(* This function block implements IEC 60870-5-101 master services *)
FUNCTION_BLOCK FB_IEC870_5_101MServices
VAR_IN_OUT
	stProcData 		: ST_IEC870_5_101MProcData;(* Process data send to or received from IEC 60870-5-101 slave device *)
	sysPara 		: ST_IEC870_5_101MSysPara; (* System parameters (data acquisition cycle times, common asdu address...) *)
	buffer			: ST_IEC870_5_101TBuffer; (* RX/TX buffer *)
	fbClock			: FB_LocalSystemTime;(* Internal clock: Local windows system time *)
	fbLog			: FB_IEC870_DebugLogFifo;(* Simple log buffer. We store/log here all our received slave data and other messages (for demonstration purpose only) *)
	bReset			: BOOL;(* Rising edge at this input resets service execution *)
END_VAR
VAR
	eState			: E_IEC870_5_101MState := e101MState_Init;(* Service/device execution state *)
	fbBuffer		: FB_IEC870_5_101TBufferCtrl;(* TX/RX buffer control function block *)
	txAsdu 			: ST_IEC870_5_101AOGen; (* Temp. asdu to send *)
	rxAsdu 			: ST_IEC870_5_101AOGen; (* Temp. received asdu *)
	
	fbTestTimer 	: TON;(* Test command cycle timer *)
	fbClockTimer	: TON;(* Clock synchronisation command cycle timer *)
	fbGeninTimer	: TON;(* General interrogation command cycle timer *)
	fbCoroTimer		: TON;(* Counter interrogation command cycle timer *)
	fbConTimer		: TON;(* Command activation confirmation timeout timer *)
	fbTermTimer		: TON;(* Command activation termination timeout timer *)
	
	bEndOfInit 		: BOOL;(* FALSE => Initialization in progress (first clock sync, general interrogation, counter interrogation... ), TRUE => End of initialization *)
	bTestConWait 	: BOOL;(* TRUE => Waiting for test command activation confirmation *)
	bClockConWait 	: BOOL;(* TRUE => Wating for clock synchronisation activation confirmation *)
	bGeninConWait	: BOOL;(* TRUE => Waiting for general interrogation activation confirmation *)
	bGeninTermWait	: BOOL;(* TRUE => Waiting for general interrogation activation termination *)
	bCoroConWait	: BOOL;(* TRUE => Waiting for counter interrogation activation confirmation *)
	bCoroTermWait	: BOOL;(* TRUE => Waiting for counter interrogation activation termination *)
	bCmdConWait		: BOOL;(* TRUE => Wating for command activation confirmation *)
	bCmdTermWait	: BOOL;(* TRUE => Waiting for command activation termination *)
	(* Temporary variables *)
	tT16			: T_CP16Time2a;(* 16 bit time tag value *)
	tT24			: T_CP24Time2a;(* 24 bit time tag value *)
	tT56			: T_CP56Time2a;(* 56 bit time tag value *)
	tT56_old		: T_CP56Time2a;(* 56 bit time tag value *)
	tT56_new		: T_CP56Time2a;(* 56 bit time tag value *)
	nCoi			: BYTE;(* Cause of initialization + LPC *)
	eCoi			: E_IEC870_5_101COI;(* Cause of initialization as enumerated type *)
	bLpc			: BOOL;(* Local parameter changed *)
	nFbp			: WORD := 16#55AA;(* Test command frame bit pattern activation data *)
	stSiq			: ST_IEC870_5_101SIQ;(* Single point information + quality descriptor *)
	stDiq			: ST_IEC870_5_101DIQ;(* Double point information + quality descriptor *)
	stQds			: ST_IEC870_5_101QDS;(* Measured value quality descriptor *)
	stQcr			: ST_IEC870_5_101QCR;(* Binary counter quality descriptor *)
	stQdp			: ST_IEC870_5_101QDP;(* Quality descriptor for events of protection equipment *)
	stSep			: ST_IEC870_5_101SEP;(* Quality descriptor for events of protection equipment *)
	stSpe			: ST_IEC870_5_101SPE;(* Start events of protection equipment *)
	stOci			: ST_IEC870_5_101OCI;(* Output cirquit information of protection equipment *)
	nVti			: BYTE;(* Value with transient state indication *)
	nBsi			: DWORD;(* Bitstring information *)
	nNva			: WORD;(* Normalized value *)
	nSva			: INT;(* Scalled value *)
	fR32			: REAL;(* Short floating point value *)
	nBcr			: DINT;(* Binary counter reading *)
	nScd			: DWORD;(* Status change detection *)
	nSco			: BYTE;(* Single command + qualifier *)
	nDco			: BYTE;(* Double  command + qualifier *)
	nRco			: BYTE;(* Regulating step command + qualifier *)
	nQos			: BYTE;(* Qualifier of setpoint command *)
	nQpm			: BYTE;(* Qualifier of parameter loading command *)
	nQpa			: BYTE;(* Qualifier of parameter activation command *)
	nQcc			: BYTE;(* Qualifier of counter interrogation command *)
	eFrz			: E_IEC870_5_101FRZ := eIEC870_FRZ_READ;
	nQoi			: BYTE;(* Qualifier of interrogation command *)
END_VAR

(* Please don't use the SIZEOF operator with CP56Time2a or CP24Time2a data type.
Because of the data alignment SIZEOF( tT56 ) or SIZEOF( tT24 ) leads to incorrect size. *)

IF bReset THEN(* Reset service execution *)
	bReset 	:= FALSE;
	eState 	:= e101MState_Init;
END_IF

(*-----------------------------------------------------------------------------------------*)
(* Generate new TX data (master requests) *)
(*-----------------------------------------------------------------------------------------*)
CASE eState OF
	e101MState_Init:(* Init state *)
		(* Reset all flags *)
		bEndOfInit 		:= FALSE;
		bTestConWait 	:= FALSE;
		bClockConWait	:= FALSE;
		bGeninConWait 	:= FALSE;
		bGeninTermWait	:= FALSE;
		bCoroConWait	:= FALSE;
		bCoroTermWait	:= FALSE;
		bCmdConWait		:= FALSE;
		bCmdTermWait	:= FALSE;
		(* Reset all timer *)
		fbTestTimer( IN := FALSE );
		fbClockTimer( IN := FALSE );
		fbGeninTimer( IN := FALSE );
		fbCoroTimer( IN := FALSE );
		fbConTimer( IN := FALSE );
		fbTermTimer( IN := FALSE );
		eState := e101MState_CycleStart;
	(*-----------------------------------------------------------------------------------------*)
	e101MState_CycleStart:(* Start of scan cycle *)
		eState := e101MState_TestAct;
	(*-----------------------------------------------------------------------------------------*)
	e101MState_TestAct:(* Send test command activation *)
		fbTestTimer( IN := bEndOfInit AND sysPara.bTest, PT := sysPara.tTest );
		IF NOT bEndOfInit OR fbTestTimer.Q THEN
			fbTestTimer( IN := FALSE );(* Reset timer *)
			fbTestTimer( IN := sysPara.bTest );
			
			(* Create asdu *)
			txAsdu.ident.eType 		:= C_TS_NA_1;(* Test command *)
			txAsdu.ident.bSQ 		:= FALSE;
			txAsdu.ident.nObj 		:= 1;
			txAsdu.ident.eCOT 		:= eIEC870_COT_ACT;(* Command activation *)
			txAsdu.ident.nORG 		:= sysPara.nOrg;(* Set originator address *)
			txAsdu.ident.bPN 		:= FALSE;
			txAsdu.ident.bT 		:= FALSE;
			txAsdu.ident.eClass 	:= eIEC870_Class_1;(* Put to the high priority tx buffer *)
			txAsdu.ident.asduAddr 	:= sysPara.asduAddr;(* Set common asdu address *)
			txAsdu.info.objAddr		:= 0;(* Set information object address *)

			nFbp := 16#55AA;(* Fixed bit pattern (FBP = 16#55AA ) to send *)
			F_iecResetStream( 0, txAsdu.info.stream );(* Clear previous data (this sets the stream length = 0 *)
			F_iecCopyBufferToStream( ADR( nFbp ), SIZEOF( nFbp ), txAsdu.info.stream );(* Put test bit pattern to stream *)
			fbBuffer.TxAddObj( putObj := txAsdu, buffer := buffer, bOk=>bTestConWait );(* Put asdu to the TX fifo *)
			IF fbBuffer.bOk THEN(* Success *)
				fbLog.A_LogHint( sPut := CONCAT( '<=', IEC101ASDU_TO_STRING( txAsdu ) ) );(* Log data (for demonstration purpose only) *)
				fbConTimer( IN := FALSE );(* Reset timer *)
				eState := e101MState_TestCon;(* Wait for test command activation confirmation *)
			ELSE(* Report send buffer overflow warning *)
				fbLog.A_LogWarning( sPut := '::TX buffer overflow (test command)!' );(* Log warning *)
			END_IF
		ELSE(* Start clock synchronisation command activation *)
			eState := e101MState_ClockAct;		
		END_IF
	
	e101MState_TestCon:(* Wait for test command activation confirmation *)
		fbConTimer( IN := bTestConWait, PT := sysPara.tCon );(* Perform timeout measure *)
		IF fbConTimer.Q THEN(* Report test command confirmation timeout error *)
			fbConTimer( IN := FALSE );(* Reset timer *)
			fbLog.A_LogError( sPut := '::Activation confirmation timeout (test command)!' );(* Log error *)
			eState := e101MState_Init;
		ELSIF NOT bTestConWait THEN(* Start clock synchronisation command activation *)
			eState := e101MState_ClockAct;
		END_IF
	(*-----------------------------------------------------------------------------------------*)
	e101MState_ClockAct:(* Send clock synchronisation command *)
		fbClockTimer( IN := bEndOfInit AND sysPara.bClock, PT := sysPara.tClock );
		IF NOT bEndOfInit OR fbClockTimer.Q THEN
			fbClockTimer( IN := FALSE );(* Reset timer *)
			fbClockTimer( IN := sysPara.bClock );
			
			(* Create asdu *)
			txAsdu.ident.eType 		:= C_CS_NA_1;(* Clock synchronisation command *)
			txAsdu.ident.bSQ 		:= FALSE;
			txAsdu.ident.nObj 		:= 1;
			txAsdu.ident.eCOT 		:= eIEC870_COT_ACT;(* Command activation *)
			txAsdu.ident.nORG 		:= sysPara.nOrg;(* Set originator address *)
			txAsdu.ident.bPN 		:= FALSE;
			txAsdu.ident.bT 		:= FALSE;
			txAsdu.ident.eClass 	:= eIEC870_Class_1;(* Put to the high priority tx buffer *)
			txAsdu.ident.asduAddr 	:= sysPara.asduAddr;(* Set common asdu address *)
			txAsdu.info.objAddr		:= 0;(* Set information object address *)
			
			tT56_new				:= SYSTEMTIME_TO_CP56Time2a( fbClock.systemTime, SU := fbClock.tzID = eTimeZoneID_Daylight );(* Get current windows loacal system time in CP56Time2a format *)
			F_iecResetStream( 0, txAsdu.info.stream );(* Clear previous data (this sets the stream length = 0 *)
			F_iecCopyBufferToStream( ADR( tT56_new ), 7(* SIZEOF( tT56_new ) - 1 *), txAsdu.info.stream );(* Put new sync time to stream *)
			fbBuffer.TxAddObj( putObj := txAsdu, buffer := buffer, bOk=>bClockConWait );(* Put asdu to the TX fifo *)
			IF fbBuffer.bOk THEN(* Success *)
				fbLog.A_LogHint( sPut := CONCAT( '<=', IEC101ASDU_TO_STRING( txAsdu ) ) );(* Log data (for demonstration purpose only) *)
				fbConTimer( IN := FALSE );(* Reset timer *)
				eState := e101MState_ClockCon;(* Wait for clock synchronisation command activation confirmation *)
			ELSE(* Report send buffer overflow warning *)
				fbLog.A_LogWarning( sPut := '::TX buffer overflow (clock synchronisation command)!' );(* Log warning *)
			END_IF			
		ELSE(* Start general interrogation command activation *)
			eState := e101MState_GeninAct;
		END_IF

	e101MState_ClockCon:(* Wait for clock synchronisation command activation confirmation *)
		fbConTimer( IN := bClockConWait, PT := sysPara.tCon );(* Perform timeout measure *)
		IF fbConTimer.Q THEN(* Report command confirmation timeout error *)
			fbConTimer( IN := FALSE );(* Reset timer *)
			fbLog.A_LogError( sPut := '::Activation confirmation timeout (clock synchronisation command)!' );(* Log error *)
			eState := e101MState_Init;
		ELSIF NOT bClockConWait THEN(* Start general interrogation command activation *)
			eState := e101MState_GeninAct;
		END_IF
	(*-----------------------------------------------------------------------------------------*)
	e101MState_GeninAct:(* Send general interrogation command activation*)
		fbGeninTimer( IN := bEndOfInit AND sysPara.bGenin, PT := sysPara.tGenin );
		IF NOT bEndOfInit OR fbGeninTimer.Q THEN
			fbGeninTimer( IN := FALSE );(* Reset timer *)
			fbGeninTimer( IN := sysPara.bGenin );
			
			(* Create asdu *)
			txAsdu.ident.eType 		:= C_IC_NA_1;(* General interrogation command *)
			txAsdu.ident.bSQ 		:= FALSE;
			txAsdu.ident.nObj 		:= 1;
			txAsdu.ident.eCOT 		:= eIEC870_COT_ACT;(* Command activation *)
			txAsdu.ident.nORG 		:= sysPara.nOrg;(* Set originator address *)
			txAsdu.ident.bPN 		:= FALSE;
			txAsdu.ident.bT 		:= FALSE;
			txAsdu.ident.eClass 	:= eIEC870_Class_1;(* Put to the high priority tx buffer *)
			txAsdu.ident.asduAddr 	:= sysPara.asduAddr;(* Set common asdu address *)
			txAsdu.info.objAddr		:= 0;(* Set information object address *)
			
			nQoi	:= INT_TO_BYTE( sysPara.eGeninQoi );(* Qualifier of general interrogation command (QOI) to send *)
			F_iecResetStream( 0, txAsdu.info.stream );(* Clear previous data (this sets the stream length = 0 *)
			F_iecCopyBufferToStream( ADR( nQoi ), SIZEOF( nQoi ), txAsdu.info.stream );(* Put QOI to stream *)
			fbBuffer.TxAddObj( putObj := txAsdu, buffer := buffer, bOk=>bGeninConWait );(* Put asdu to the TX fifo *)
			IF fbBuffer.bOk THEN(* Success *)
				fbLog.A_LogHint( sPut := CONCAT( '<=', IEC101ASDU_TO_STRING( txAsdu ) ) );(* Log data (for demonstration purpose only) *)
				fbConTimer( IN := FALSE );(* Reset timer *)
				fbTermTimer( IN := FALSE );(* Reset timer *)
				bGeninTermWait := bGeninConWait;(* Wait for general interrogation activation termination too *)
				eState := e101MState_GeninCon;(* Wait for general interrogation activation confirmation *)
			ELSE(* Report send buffer overflow warning  *)
				fbLog.A_LogWarning( sPut := '::TX buffer overflow (general interrogation command)!' );(* Log warning *)
			END_IF
		ELSE(* Start counter interrogation command activation *)
			eState := e101MState_Coro;
		END_IF

	e101MState_GeninCon:(* Wait for general interrogation command activation confirmation *)
		fbConTimer( IN := bGeninConWait, PT := sysPara.tCon );(* Perform timeout measure *)
		IF fbConTimer.Q THEN(* Report general interrogation command activation confirmation timeout error *)
			fbConTimer( IN := FALSE );(* Reset timer *)
			fbLog.A_LogError( sPut := '::Activation confirmation timeout (general interrogation command)!' );(* Log error *)
			eState := e101MState_Init;
		ELSIF NOT bGeninConWait THEN(* Wait for general interrogation activation termination *)
			eState := e101MState_GeninTerm;
		END_IF
		
	e101MState_GeninTerm:(* Wait for general interrogation command activation termination *)
		fbTermTimer( IN := bGeninTermWait, PT := sysPara.tTerm );(* Perform timeout measure *)
		IF fbTermTimer.Q THEN(* Report general interrogation command activation termination timeout error *)
			fbTermTimer( IN := FALSE );(* Reset timer *)
			fbLog.A_LogError( sPut := '::Activation termination timeout (general interrogation command)!' );(* Log error *)
			eState := e101MState_Init;
		ELSIF NOT bGeninTermWait THEN(* Start counter interrogation command activation *)
			eState := e101MState_Coro;
		END_IF
	(*-----------------------------------------------------------------------------------------*)
	e101MState_Coro:(* Counter interrogation *)
		fbCoroTimer( IN := bEndOfInit AND sysPara.bCoro, PT := sysPara.tCoro );
		IF NOT bEndOfInit OR fbCoroTimer.Q THEN
			fbCoroTimer( IN := FALSE );(* Reset timer *)
			fbCoroTimer( IN := sysPara.bCoro );
			IF ( sysPara.eCoroMode = eIEC870_CoroMode_A ) THEN
				eState := e101MState_CmdAct;(* Do nothing *)
			ELSIF ( sysPara.eCoroMode = eIEC870_CoroMode_B ) THEN
				eState := e101MState_CoroReadAct;(* Read only *)			
			ELSIF ( sysPara.eCoroMode = eIEC870_CoroMode_C ) THEN
				eState := e101MState_CoroFrzRstAct;(* Freeze and/or reset first and then read *)			
			ELSIF ( sysPara.eCoroMode = eIEC870_CoroMode_D ) THEN
				eState := e101MState_CoroFrzRstAct;(* Freeze and/or reset only *)			
			END_IF
		ELSE(* Start single/double command activation *)
			eState := e101MState_CmdAct;
		END_IF
	(*-----------------------------------------------------------------------------------------*)
	e101MState_CoroFrzRstAct:(* Send counter freeze and/or reset command *)
		(* Create asdu *)
		txAsdu.ident.eType 		:= C_CI_NA_1;(* Counter interrogation command *)
		txAsdu.ident.bSQ 		:= FALSE;
		txAsdu.ident.nObj 		:= 1;
		txAsdu.ident.eCOT 		:= eIEC870_COT_ACT;(* Command activation *)
		txAsdu.ident.nORG 		:= sysPara.nOrg;(* Set originator address *)
		txAsdu.ident.bPN 		:= FALSE;
		txAsdu.ident.bT 		:= FALSE;
		txAsdu.ident.eClass 	:= eIEC870_Class_1;(* Put to the high priority tx buffer *)
		txAsdu.ident.asduAddr 	:= sysPara.asduAddr;(* Set common asdu address *)
		txAsdu.info.objAddr		:= 0;(* Set information object address *)
	
		eFrz := SEL( sysPara.bCoroReset, eIEC870_FRZ_FREEZE, eIEC870_FRZ_FREEZE_AND_RESET );
		nQcc := SHL( INT_TO_BYTE( eFrz ), 6 ) OR INT_TO_BYTE( sysPara.eCoroRqt );(* Create qualifier of counter interrogation command (QCC) *)
		
		F_iecResetStream( 0, txAsdu.info.stream );(* Clear previous data (this sets the stream length = 0 *)
		F_iecCopyBufferToStream( ADR( nQcc ), SIZEOF( nQcc ), txAsdu.info.stream );(* Put QCC to stream *)
		fbBuffer.TxAddObj( putObj := txAsdu, buffer := buffer, bOk=>bCoroConWait );(* Put asdu to the TX fifo *)
		IF fbBuffer.bOk THEN(* Success *)
			fbLog.A_LogHint( sPut := CONCAT( '<=', IEC101ASDU_TO_STRING( txAsdu ) ) );(* Log data (for demonstration purpose only) *)
			fbConTimer( IN := FALSE );(* Reset timer *)
			eState := e101MState_CoroFrzRstCon;(* Wait for counter interrogation command activation confirmation *)
		ELSE(* Report send buffer overflow warning *)
			fbLog.A_LogWarning( sPut := '::TX buffer overflow (counter interrogation command)!' );(* Log warning *)
		END_IF
		
	e101MState_CoroFrzRstCon:(* Wait for counter interrogation command activation confirmation *)
		fbConTimer( IN := bCoroConWait, PT := sysPara.tCon );(* Perform timeout measure *)
		IF fbConTimer.Q THEN(* Report command activation confirmation timeout error *)
			fbConTimer( IN := FALSE );(* Reset timer *)
			fbLog.A_LogError( sPut := '::Activation confirmation timeout (counter interrogation command)!' );(* Log error *)
			eState := e101MState_Init;
		ELSIF NOT bCoroConWait THEN
			IF sysPara.eCoroMode = eIEC870_CoroMode_C THEN
				eState := e101MState_CoroReadAct;
			ELSE(* Mode D *)
				eState := e101MState_Init;
			END_IF			
		END_IF
		
	(*-----------------------------------------------------------------------------------------*)
	e101MState_CoroReadAct:(* Send counter read command *)
		(* Create asdu *)
		txAsdu.ident.eType 		:= C_CI_NA_1;(* Counter interrogation command *)
		txAsdu.ident.bSQ 		:= FALSE;
		txAsdu.ident.nObj 		:= 1;
		txAsdu.ident.eCOT 		:= eIEC870_COT_ACT;(* Command activation *)
		txAsdu.ident.nORG 		:= sysPara.nOrg;(* Set originator address *)
		txAsdu.ident.bPN 		:= FALSE;
		txAsdu.ident.bT 		:= FALSE;
		txAsdu.ident.eClass 	:= eIEC870_Class_1;(* Put to the high priority tx buffer *)
		txAsdu.ident.asduAddr 	:= sysPara.asduAddr;(* Set common asdu address *)
		txAsdu.info.objAddr		:= 0;(* Set information object address *)
		
		eFrz := eIEC870_FRZ_READ;
		nQcc	:= SHL( INT_TO_BYTE( eFRZ ), 6 ) OR INT_TO_BYTE( sysPara.eCoroRqt );(* Create qualifier of counter interrogation command (QCC) *)
		
		F_iecResetStream( 0, txAsdu.info.stream );(* Clear previous data (this sets the stream length = 0 *)
		F_iecCopyBufferToStream( ADR( nQcc ), SIZEOF( nQcc ), txAsdu.info.stream );(* Put QCC to stream *)
		fbBuffer.TxAddObj( putObj := txAsdu, buffer := buffer, bOk=>bCoroConWait );(* Put asdu to the TX fifo *)
		IF fbBuffer.bOk THEN(* Success *)
			fbLog.A_LogHint( sPut := CONCAT( '<=', IEC101ASDU_TO_STRING( txAsdu ) ) );(* Log data (for demonstration purpose only) *)
			fbConTimer( IN := FALSE );(* Reset timer *)
			fbTermTimer( IN := FALSE );(* Reset timer *)
			bCoroTermWait := bCoroConWait;(* Wait for counter interrogation activation termination too *)
			eState := e101MState_CoroReadCon;(* Wait for counter interrogation command activation confirmation *)
		ELSE(* Report send buffer overflow warning *)
			fbLog.A_LogWarning( sPut := '::TX buffer overflow (counter interrogation command)!' );(* Log warning *)
		END_IF
	
	e101MState_CoroReadCon:(* Wait for counter interrogation command activation confirmation *)
		fbConTimer( IN := bCoroConWait, PT := sysPara.tCon );(* Perform timeout measure *)
		IF fbConTimer.Q THEN(* Report command activation confirmation timeout error *)
			fbConTimer( IN := FALSE );(* Reset timer *)
			fbLog.A_LogError( sPut := '::Activation confirmation timeout (counter interrogation command)!' );(* Log error *)
			eState := e101MState_Init;
		ELSIF NOT bCoroConWait THEN(* Wait for counter interrogation command activation termination *)
			eState := e101MState_CoroReadTerm;
		END_IF

	e101MState_CoroReadTerm:(* Wait for counter interrogation command activation termination *)
		fbTermTimer( IN := bCoroTermWait, PT := sysPara.tTerm );(* Perform timeout measure *)
		IF fbTermTimer.Q THEN(* Report counter interrogation command activation termination timeout error *)
			fbTermTimer( IN := FALSE );(* Reset timer *)
			fbLog.A_LogError( sPut := '::Activation termination timeout (counter interrogation command)!' );(* Log error *)
			eState := e101MState_Init;
		ELSIF NOT bCoroTermWait THEN(* Start single/double point command activation *)
			eState := e101MState_CmdAct;
		END_IF
	(*-----------------------------------------------------------------------------------------*)
	(*############################ COMMAND EXECUTION ##########################################*)
	(*-----------------------------------------------------------------------------------------*)
	e101MState_CmdAct:(* Send command(s) *)
		IF stProcData.eCtrl10 <> eIEC870_CMD_NONE THEN(* Send single command activation*)
			
			(* Create asdu *)
			txAsdu.ident.eType 		:= C_SC_NA_1;(* Single command *)
			txAsdu.ident.bSQ 		:= FALSE;
			txAsdu.ident.nObj 		:= 1;
			txAsdu.ident.eCOT 		:= SEL( stProcData.eCtrl10 = eIEC870_CMD_DESELECT, eIEC870_COT_ACT, eIEC870_COT_DEACT );(* Command activation/deactivation *)
			txAsdu.ident.nORG 		:= sysPara.nOrg;(* Set originator address *)
			txAsdu.ident.bPN 		:= FALSE;
			txAsdu.ident.bT 		:= FALSE;
			txAsdu.ident.eClass 	:= eIEC870_Class_1;(* Put to the high priority tx buffer *)
			txAsdu.ident.asduAddr 	:= sysPara.asduAddr;(* Set common asdu address *)
			txAsdu.info.objAddr		:= 10;(* Set information object address *)

			nSco 	:= SHL( INT_TO_BYTE( stProcData.eQu10 ), 2 ) OR INT_TO_BYTE( stProcData.eScs10 );(* Set single command qualifier + state *)
			nSco.7 	:= ( stProcData.eCtrl10 = eIEC870_CMD_SELECT );(* Set select/execute bit (1 := select, 0:= execute *)
			
			F_iecResetStream( 0, txAsdu.info.stream );(* Clear previous data (this sets the stream length = 0 *)
			F_iecCopyBufferToStream( ADR( nSco ), SIZEOF( nSco ), txAsdu.info.stream );(* Put QCC to stream *)
			fbBuffer.TxAddObj( putObj := txAsdu, buffer := buffer, bOk=>bCmdConWait );(* Put asdu to the TX fifo *)
			IF fbBuffer.bOk THEN(* Success *)
				fbLog.A_LogHint( sPut := CONCAT( '<=', IEC101ASDU_TO_STRING( txAsdu ) ) );(* Log data (for demonstration purpose only) *)
				fbConTimer( IN := FALSE );(* Reset timer *)
				fbTermTimer( IN := FALSE );(* Reset timer *)
				bCmdTermWait := NOT ( stProcData.eCtrl10 = eIEC870_CMD_SELECT );(* If EXECUTE (direct) command => Wait for activation termination *)
				stProcData.eCtrl10 := eIEC870_CMD_NONE;(* Disable command execution *)
				eState := e101MState_CmdCon;(* Wait for command activation confirmation *)
			ELSE(* Report send buffer overflow warning *)
				fbLog.A_LogWarning( sPut := '::TX buffer overflow (single command)!' );(* Log warning *)
			END_IF

		ELSIF stProcData.eCtrl20 <> eIEC870_CMD_NONE THEN(* Send double command activation *)
			
			(* Create asdu *)
			txAsdu.ident.eType 		:= C_DC_NA_1;(* Double command *)
			txAsdu.ident.bSQ 		:= FALSE;
			txAsdu.ident.nObj 		:= 1;
			txAsdu.ident.eCOT 		:= SEL( stProcData.eCtrl20 = eIEC870_CMD_DESELECT, eIEC870_COT_ACT, eIEC870_COT_DEACT );(* Command activation/deactivation *)
			txAsdu.ident.nORG 		:= sysPara.nOrg;(* Set originator address *)
			txAsdu.ident.bPN 		:= FALSE;
			txAsdu.ident.bT 		:= FALSE;
			txAsdu.ident.eClass 	:= eIEC870_Class_1;(* Put to the high priority tx buffer *)
			txAsdu.ident.asduAddr 	:= sysPara.asduAddr;(* Set common asdu address *)
			txAsdu.info.objAddr		:= 20;(* Set information object address *)
			
			nDco	:= SHL( INT_TO_BYTE( stProcData.eQu20 ), 2 ) OR INT_TO_BYTE( stProcData.eDcs20 );(* Set double command qualifier + state *)
			nDco.7 	:= ( stProcData.eCtrl20 = eIEC870_CMD_SELECT );(* Set select/execute bit *)
			
			F_iecResetStream( 0, txAsdu.info.stream );(* Clear previous data (this sets the stream length = 0 *)
			F_iecCopyBufferToStream( ADR( nDco ), SIZEOF( nDco ), txAsdu.info.stream );(* Put QCC to stream *)
			fbBuffer.TxAddObj( putObj := txAsdu, buffer := buffer, bOk=>bCmdConWait );(* Put asdu to the TX fifo *)
			IF fbBuffer.bOk THEN(* Success *)
				fbLog.A_LogHint( sPut := CONCAT( '<=', IEC101ASDU_TO_STRING( txAsdu ) ) );(* Log data (for demonstration purpose only) *)
				fbConTimer( IN := FALSE );(* Reset timer *)
				fbTermTimer( IN := FALSE );(* Reset timer *)
				bCmdTermWait := NOT ( stProcData.eCtrl20 = eIEC870_CMD_SELECT );(* If EXECUTE (direct) command => Wait for activation termination *)
				stProcData.eCtrl20 := eIEC870_CMD_NONE;(* Disable command execution *)
				eState := e101MState_CmdCon;(* Wait for command activation confirmation *)
			ELSE(* Report send buffer overflow warning *)
				fbLog.A_LogWarning( sPut := '::TX buffer overflow (double command)!' );(* Log warning*)
			END_IF
			
		ELSIF stProcData.eCtrl30 <> eIEC870_CMD_NONE THEN(* Send regulating step command activation*)
			
			(* Create asdu *)
			txAsdu.ident.eType 		:= C_RC_NA_1;(* Regulating step command *)
			txAsdu.ident.bSQ 		:= FALSE;
			txAsdu.ident.nObj 		:= 1;
			txAsdu.ident.eCOT 		:= SEL( stProcData.eCtrl30 = eIEC870_CMD_DESELECT, eIEC870_COT_ACT, eIEC870_COT_DEACT );(* Command activation/deactivation *)
			txAsdu.ident.nORG 		:= sysPara.nOrg;(* Set originator address *)
			txAsdu.ident.bPN 		:= FALSE;
			txAsdu.ident.bT 		:= FALSE;
			txAsdu.ident.eClass 	:= eIEC870_Class_1;(* Put to the high priority tx buffer *)
			txAsdu.ident.asduAddr 	:= sysPara.asduAddr;(* Set common asdu address *)
			txAsdu.info.objAddr		:= 30;(* Set information object address *)
			
			nRco	:= SHL( INT_TO_BYTE( stProcData.eQu30 ), 2 ) OR INT_TO_BYTE( stProcData.eRcs30 );(* Set regulating step command qualifier + state *)
			nRco.7 	:= ( stProcData.eCtrl30 = eIEC870_CMD_SELECT );(* Set select/execute bit *)
			
			F_iecResetStream( 0, txAsdu.info.stream );(* Clear previous data (this sets the stream length = 0 *)
			F_iecCopyBufferToStream( ADR( nRco ), SIZEOF( nRco ), txAsdu.info.stream );(* Put RCO to stream *)
			fbBuffer.TxAddObj( putObj := txAsdu, buffer := buffer, bOk=>bCmdConWait );(* Put asdu to the TX fifo *)
			IF fbBuffer.bOk THEN(* Success *)
				fbLog.A_LogHint( sPut := CONCAT( '<=', IEC101ASDU_TO_STRING( txAsdu ) ) );(* Log data (for demonstration purpose only) *)
				fbConTimer( IN := FALSE );(* Reset timer *)
				fbTermTimer( IN := FALSE );(* Reset timer *)
				bCmdTermWait := NOT ( stProcData.eCtrl30 = eIEC870_CMD_SELECT );(* If EXECUTE (direct) command => Wait for activation termination *)
				stProcData.eCtrl30 := eIEC870_CMD_NONE;(* Disable command execution *)
				eState := e101MState_CmdCon;(* Wait for command activation confirmation *)
			ELSE(* Report send buffer overflow warning *)
				fbLog.A_LogWarning( sPut := '::TX buffer overflow (regulating step command)!' );(* Log warning*)
			END_IF
			
		ELSIF stProcData.eCtrl40 <> eIEC870_CMD_NONE THEN(* Send bitstring command activation*)

			(* Create asdu *)
			txAsdu.ident.eType 		:= C_BO_NA_1;(* Bitstring command *)
			txAsdu.ident.bSQ 		:= FALSE;
			txAsdu.ident.nObj 		:= 1;
			txAsdu.ident.eCOT 		:= SEL( stProcData.eCtrl40 = eIEC870_CMD_DESELECT, eIEC870_COT_ACT, eIEC870_COT_DEACT );(* Command activation/deactivation *)
			txAsdu.ident.nORG 		:= sysPara.nOrg;(* Set originator address *)
			txAsdu.ident.bPN 		:= FALSE;
			txAsdu.ident.bT 		:= FALSE;
			txAsdu.ident.eClass 	:= eIEC870_Class_1;(* Put to the high priority tx buffer *)
			txAsdu.ident.asduAddr 	:= sysPara.asduAddr;(* Set common asdu address *)
			txAsdu.info.objAddr		:= 40;(* Set information object address *)
			
			nBsi	:= stProcData.nBsi40;(* Set BSI value *)
			
			F_iecResetStream( 0, txAsdu.info.stream );(* Clear previous data (this sets the stream length = 0 *)
			F_iecCopyBufferToStream( ADR( nBsi ), SIZEOF( nBsi ), txAsdu.info.stream );(* Put BSI to stream *)
			fbBuffer.TxAddObj( putObj := txAsdu, buffer := buffer, bOk=>bCmdConWait );(* Put asdu to the TX fifo *)
			IF fbBuffer.bOk THEN(* Success *)
				fbLog.A_LogHint( sPut := CONCAT( '<=', IEC101ASDU_TO_STRING( txAsdu ) ) );(* Log data (for demonstration purpose only) *)
				fbConTimer( IN := FALSE );(* Reset timer *)
				stProcData.eCtrl40 := eIEC870_CMD_NONE;(* Disable command execution *)
				eState := e101MState_CmdCon;(* Wait for command activation confirmation *)
			ELSE(* Report send buffer overflow warning *)
				fbLog.A_LogWarning( sPut := '::TX buffer overflow (bitstring command)!' );(* Log warning*)
			END_IF

		ELSIF stProcData.eCtrl50 <> eIEC870_CMD_NONE THEN(* Send setpoint command activation, normalized value *)

			(* Create asdu *)
			txAsdu.ident.eType 		:= C_SE_NA_1;(* Setpoint command, normalized value*)
			txAsdu.ident.bSQ 		:= FALSE;
			txAsdu.ident.nObj 		:= 1;
			txAsdu.ident.eCOT 		:= SEL( stProcData.eCtrl50 = eIEC870_CMD_DESELECT, eIEC870_COT_ACT, eIEC870_COT_DEACT );(* Command activation/deactivation *)
			txAsdu.ident.nORG 		:= sysPara.nOrg;(* Set originator address *)
			txAsdu.ident.bPN 		:= FALSE;
			txAsdu.ident.bT 		:= FALSE;
			txAsdu.ident.eClass 	:= eIEC870_Class_1;(* Put to the high priority tx buffer *)
			txAsdu.ident.asduAddr 	:= sysPara.asduAddr;(* Set common asdu address *)
			txAsdu.info.objAddr		:= 50;(* Set information object address *)
			
			nNva	:= stProcData.nNva50;(* Set NVA value *)
			nQos	:= INT_TO_BYTE( stProcData.eQl50 );(* Set qualifier of command *)
			nQos.7 	:= stProcData.eCtrl50 = eIEC870_CMD_SELECT;(* Set select/execute bit *)
			
			F_iecResetStream( 0, txAsdu.info.stream );(* Clear previous data (this sets the stream length = 0 *)
			F_iecCopyBufferToStream( ADR( nNva ), SIZEOF( nNva ), txAsdu.info.stream );(* Put NVA to stream *)
			F_iecCopyBufferToStream( ADR( nQos ), SIZEOF( nQos ), txAsdu.info.stream );(* Put QOS to stream *)
			fbBuffer.TxAddObj( putObj := txAsdu, buffer := buffer, bOk=>bCmdConWait );(* Put asdu to the TX fifo *)
			IF fbBuffer.bOk THEN(* Success *)
				fbLog.A_LogHint( sPut := CONCAT( '<=', IEC101ASDU_TO_STRING( txAsdu ) ) );(* Log data (for demonstration purpose only) *)
				fbConTimer( IN := FALSE );(* Reset timer *)
				stProcData.eCtrl50 := eIEC870_CMD_NONE;(* Disable command execution *)
				eState := e101MState_CmdCon;(* Wait for command activation confirmation *)
			ELSE(* Report send buffer overflow warning *)
				fbLog.A_LogWarning( sPut := '::TX buffer overflow (setpoint command, normalized value)!' );(* Log warning*)
			END_IF

		ELSIF stProcData.eCtrl60 <> eIEC870_CMD_NONE THEN(* Send setpoint, scalled value command activation*)

			(* Create asdu *)
			txAsdu.ident.eType 		:= C_SE_NB_1;(* Setpoint command, scalled value*)
			txAsdu.ident.bSQ 		:= FALSE;
			txAsdu.ident.nObj 		:= 1;
			txAsdu.ident.eCOT 		:= SEL( stProcData.eCtrl60 = eIEC870_CMD_DESELECT, eIEC870_COT_ACT, eIEC870_COT_DEACT );(* Command activation/deactivation *)
			txAsdu.ident.nORG 		:= sysPara.nOrg;(* Set originator address *)
			txAsdu.ident.bPN 		:= FALSE;
			txAsdu.ident.bT 		:= FALSE;
			txAsdu.ident.eClass 	:= eIEC870_Class_1;(* Put to the high priority tx buffer *)
			txAsdu.ident.asduAddr 	:= sysPara.asduAddr;(* Set common asdu address *)
			txAsdu.info.objAddr		:= 60;(* Set information object address *)
			
			nSva	:= stProcData.nSva60;(* Set SVA value *)
			nQos	:= INT_TO_BYTE( stProcData.eQl60 );(* Set qualifier of command *)
			nQos.7 	:= stProcData.eCtrl60 = eIEC870_CMD_SELECT;(* Set select/execute bit *)
			
			F_iecResetStream( 0, txAsdu.info.stream );(* Clear previous data (this sets the stream length = 0 *)
			F_iecCopyBufferToStream( ADR( nSva ), SIZEOF( nSva ), txAsdu.info.stream );(* Put SVA to stream *)
			F_iecCopyBufferToStream( ADR( nQos ), SIZEOF( nQos ), txAsdu.info.stream );(* Put QOS to stream *)
			fbBuffer.TxAddObj( putObj := txAsdu, buffer := buffer, bOk=>bCmdConWait );(* Put asdu to the TX fifo *)
			IF fbBuffer.bOk THEN(* Success *)
				fbLog.A_LogHint( sPut := CONCAT( '<=', IEC101ASDU_TO_STRING( txAsdu ) ) );(* Log data (for demonstration purpose only) *)
				fbConTimer( IN := FALSE );(* Reset timer *)
				stProcData.eCtrl60 := eIEC870_CMD_NONE;(* Disable command execution *)
				eState := e101MState_CmdCon;(* Wait for command activation confirmation *)
			ELSE(* Report send buffer overflow warning *)
				fbLog.A_LogWarning( sPut := '::TX buffer overflow (setpoint command, scalled value)!' );(* Log warning*)
			END_IF

		ELSIF stProcData.eCtrl70 <> eIEC870_CMD_NONE THEN(* Send setpoint, short floating point value command activation*)

			(* Create asdu *)
			txAsdu.ident.eType 		:= C_SE_NC_1;(* Setpoint command, short floating point value*)
			txAsdu.ident.bSQ 		:= FALSE;
			txAsdu.ident.nObj 		:= 1;
			txAsdu.ident.eCOT 		:= SEL( stProcData.eCtrl70 = eIEC870_CMD_DESELECT, eIEC870_COT_ACT, eIEC870_COT_DEACT );(* Command activation/deactivation *)
			txAsdu.ident.nORG 		:= sysPara.nOrg;(* Set originator address *)
			txAsdu.ident.bPN 		:= FALSE;
			txAsdu.ident.bT 		:= FALSE;
			txAsdu.ident.eClass 	:= eIEC870_Class_1;(* Put to the high priority tx buffer *)
			txAsdu.ident.asduAddr 	:= sysPara.asduAddr;(* Set common asdu address *)
			txAsdu.info.objAddr		:= 70;(* Set information object address *)
			
			fR32	:= stProcData.fSingle70;(* Set R32 value *)
			nQos	:= INT_TO_BYTE( stProcData.eQl70 );(* Set qualifier of command *)
			nQos.7 	:= stProcData.eCtrl70 = eIEC870_CMD_SELECT;(* Set select/execute bit *)
			
			F_iecResetStream( 0, txAsdu.info.stream );(* Clear previous data (this sets the stream length = 0 *)
			F_iecCopyBufferToStream( ADR( fR32 ), SIZEOF( fR32 ), txAsdu.info.stream );(* Put R32 to stream *)
			F_iecCopyBufferToStream( ADR( nQos ), SIZEOF( nQos ), txAsdu.info.stream );(* Put QOS to stream *)
			fbBuffer.TxAddObj( putObj := txAsdu, buffer := buffer, bOk=>bCmdConWait );(* Put asdu to the TX fifo *)
			IF fbBuffer.bOk THEN(* Success *)
				fbLog.A_LogHint( sPut := CONCAT( '<=', IEC101ASDU_TO_STRING( txAsdu ) ) );(* Log data (for demonstration purpose only) *)
				fbConTimer( IN := FALSE );(* Reset timer *)
				stProcData.eCtrl70 := eIEC870_CMD_NONE;(* Disable command execution *)
				eState := e101MState_CmdCon;(* Wait for command activation confirmation *)
			ELSE(* Report send buffer overflow warning *)
				fbLog.A_LogWarning( sPut := '::TX buffer overflow (setpoint command, short floating point value)!' );(* Log warning*)
			END_IF

		ELSE(* End of scan cycle *)
			eState := e101MState_CycleEnd;
		END_IF
	(*-----------------------------------------------------------------------------------------*)
	(*#########################################################################################*)
	(*-----------------------------------------------------------------------------------------*)
	e101MState_CmdCon:(* Wait for single-point/double-point/setpoint command activation confirmation *)
		fbConTimer( IN := bCmdConWait, PT := sysPara.tCon );(* Perform timeout measure *)
		IF fbConTimer.Q THEN(* Report command activation confirmation timeout error *)
			fbConTimer( IN := FALSE );(* Reset timer *)
			fbLog.A_LogError( sPut := '::Activation confirmation timeout (single/double command)!' );(* Log error *)
			eState := e101MState_Init;
		ELSIF NOT bCmdConWait THEN(* Wait for command activation termination *)
			eState := e101MState_CmdTerm;
		END_IF
	(*-----------------------------------------------------------------------------------------*)
	e101MState_CmdTerm:(* Wait for single-point/double-point/setpoint command activation termination *)
		fbTermTimer( IN := bCmdTermWait, PT := sysPara.tTerm );(* Perform timeout measure *)
		IF fbTermTimer.Q THEN(* Report command activation termination timeout error *)
			fbTermTimer( IN := FALSE );(* Reset timer *)
			fbLog.A_LogError( sPut := '::Activation termination timeout (single/double command)!' );(* Log error *)
			eState := e101MState_Init;
		ELSIF NOT bCmdTermWait THEN(* End of scan cycle *)
			eState := e101MState_CycleEnd;
		END_IF
	(*-----------------------------------------------------------------------------------------*)
	e101MState_CycleEnd:(* End of scan cycle *)
		bEndOfInit := TRUE;(* Set init flag *)
		eState := e101MState_CycleStart;(* Repeat polling cycle (acquisition of data)*)

ELSE(* Fatal error *)
	fbLog.A_LogError( sPut := '::Fatal error (invalid state)!' );
	eState := e101MState_Init;	
END_CASE



(*-----------------------------------------------------------------------------------------*)
(* Interpret RX data (slave responses) *)
(*-----------------------------------------------------------------------------------------*)
REPEAT
	fbBuffer.RxRemoveObj( getObj=>rxAsdu, buffer := buffer ); (* Try to remove asdu from RX fifo *)
	IF fbBuffer.bOk THEN (* Success *)

		fbLog.A_LogHint( sPut := CONCAT( '=>', IEC101ASDU_TO_STRING( rxAsdu ) ) );(* Log data (for demonstration purpose only) *)

		CASE rxAsdu.ident.eType OF
			(*-----------------------------------------------------------------------------------------*)
			C_TS_NA_1: (* Test command activation confirmation *)
				F_iecMoveStreamToBuffer( ADR( nFbp ), SIZEOF( nFbp ), rxAsdu.info.stream );(* Copy the returned FBP to local variable *)
				IF nFbp <> 16#55AA THEN(* Report test command error *)
					fbLog.A_LogError( sPut := '::Test command error (invalid FBP)!' );
				END_IF
				IF rxAsdu.ident.eCOT = eIEC870_COT_ACT_CON THEN
					bTestConWait := FALSE;(* Reset wait flag *)
				END_IF
			(*-----------------------------------------------------------------------------------------*)
			C_CS_NA_1: (* Clock synchronisation command activation confirmation *)
				F_iecMoveStreamToBuffer( ADR( tT56_old ), 7(* SIZEOF( tT56_old ) - 1 *), rxAsdu.info.stream );(* Copy returned old server time to local variable *)
				IF rxAsdu.ident.eCOT = eIEC870_COT_ACT_CON THEN
					bClockConWait := FALSE;(* Reset wait flag *)
				END_IF
			(*-----------------------------------------------------------------------------------------*)
			C_IC_NA_1: (* General interrogation command activation confirmation/termination *)
				F_iecMoveStreamToBuffer( ADR( nQoi ), SIZEOF( nQoi ), rxAsdu.info.stream );(* Copy returned QOI to local variable *)
				IF rxAsdu.ident.eCOT = eIEC870_COT_ACT_CON THEN
					bGeninConWait := FALSE;(* Reset wait flag *)
				END_IF
				IF rxAsdu.ident.eCOT = eIEC870_COT_ACT_TERM THEN
					bGeninTermWait := FALSE;(* Reset wait flag *)
				END_IF
			(*-----------------------------------------------------------------------------------------*)
			C_CI_NA_1: (* Counter interrogation command activation confirmation/termination *)
				F_iecMoveStreamToBuffer( ADR( nQcc ), SIZEOF( nQcc ), rxAsdu.info.stream );(* Copy returned QCC to local variable *)
				IF rxAsdu.ident.eCOT = eIEC870_COT_ACT_CON THEN
					bCoroConWait := FALSE;(* Reset wait flag *)
				END_IF
				IF rxAsdu.ident.eCOT = eIEC870_COT_ACT_TERM THEN(* Optional *)
					bCoroTermWait := FALSE;(* Reset wait flag *)
				END_IF
			(*-----------------------------------------------------------------------------------------*)
			M_SP_NA_1, M_SP_TA_1, M_SP_TB_1:(* Single points *)
				F_iecMoveStreamToBuffer( ADR( stSiq ), SIZEOF( stSiq ), rxAsdu.info.stream );(* Copy SIQ to local variable *)
				IF rxAsdu.ident.eType = M_SP_TA_1 THEN
					F_iecMoveStreamToBuffer( ADR( tT24 ), 3(* SIZEOF( tT24 ) - 1 *), rxAsdu.info.stream );(* Copy time tag to local variable *)
				ELSIF rxAsdu.ident.eType = M_SP_TB_1 THEN
					F_iecMoveStreamToBuffer( ADR( tT56 ), 7(* SIZEOF( tT56 ) - 1 *), rxAsdu.info.stream );(* Copy time tag to local variable *)
				END_IF
				IF rxAsdu.info.objAddr = 100 THEN
					stProcData.stSiq100 := stSiq;
				ELSIF rxAsdu.info.objAddr = 101 THEN
					stProcData.stSiq101 := stSiq;
				ELSIF rxAsdu.info.objAddr = 102 THEN
					stProcData.stSiq102 := stSiq;
				END_IF
			(*-----------------------------------------------------------------------------------------*)
			M_DP_NA_1, M_DP_TA_1, M_DP_TB_1:(* Double points *)
				F_iecMoveStreamToBuffer( ADR( stDiq ), SIZEOF( stDiq ), rxAsdu.info.stream );(* Copy DIQ to local variable *)
				IF rxAsdu.ident.eType = M_DP_TA_1 THEN
					F_iecMoveStreamToBuffer( ADR( tT24 ), 3(* SIZEOF( tT24 ) - 1 *), rxAsdu.info.stream );(* Copy time tag to local variable *)
				ELSIF rxAsdu.ident.eType = M_DP_TB_1 THEN
					F_iecMoveStreamToBuffer( ADR( tT56 ), 7(* SIZEOF( tT56 ) - 1 *), rxAsdu.info.stream );(* Copy time tag to local variable *)
				END_IF
				IF rxAsdu.info.objAddr = 200 THEN
					stProcData.stDiq200 := stDiq; 
				END_IF
			(*-----------------------------------------------------------------------------------------*)
			M_ST_NA_1, M_ST_TA_1, M_ST_TB_1:(* Regulating step values *)
				F_iecMoveStreamToBuffer( ADR( nVti ), SIZEOF( nVti ), rxAsdu.info.stream );(* Copy VTI to local variable *)
				F_iecMoveStreamToBuffer( ADR( stQds ), SIZEOF( stQds ), rxAsdu.info.stream );(* Copy QDS to local variable *)
				IF rxAsdu.ident.eType = M_ST_TA_1 THEN
					F_iecMoveStreamToBuffer( ADR( tT24 ), 3(* SIZEOF( tT24 ) - 1 *), rxAsdu.info.stream );(* Copy time tag to local variable *)
				ELSIF rxAsdu.ident.eType = M_ST_TB_1 THEN
					F_iecMoveStreamToBuffer( ADR( tT56 ), 7(* SIZEOF( tT56 ) - 1 *), rxAsdu.info.stream );(* Copy time tag to local variable *)
				END_IF
				IF rxAsdu.info.objAddr = 300 THEN
					stProcData.nVti300 := nVti; 
					stProcData.stQds300 := stQds; 
				END_IF
			(*-----------------------------------------------------------------------------------------*)
			M_BO_NA_1, M_BO_TA_1, M_BO_TB_1:(* Bitstring values *)
				F_iecMoveStreamToBuffer( ADR( nBsi ), SIZEOF( nBsi ), rxAsdu.info.stream );(* Copy BSI to local variable *)
				F_iecMoveStreamToBuffer( ADR( stQds ), SIZEOF( stQds ), rxAsdu.info.stream );(* Copy QDS to local variable *)
				IF rxAsdu.ident.eType = M_BO_TA_1 THEN
					F_iecMoveStreamToBuffer( ADR( tT24 ), 3(* SIZEOF( tT24 ) - 1 *), rxAsdu.info.stream );(* Copy time tag to local variable *)
				ELSIF rxAsdu.ident.eType = M_BO_TB_1 THEN
					F_iecMoveStreamToBuffer( ADR( tT56 ), 7(* SIZEOF( tT56 ) - 1 *), rxAsdu.info.stream );(* Copy time tag to local variable *)
				END_IF
				IF rxAsdu.info.objAddr = 400 THEN 
					stProcData.nBsi400 := nBsi;
					stProcData.stQds400 := stQds;
				END_IF
			(*-----------------------------------------------------------------------------------------*)
			M_ME_NA_1, M_ME_TA_1, M_ME_TD_1, M_ME_ND_1:(* Measured values, normalized values *)
				F_iecMoveStreamToBuffer( ADR( nNva ), SIZEOF( nNva ), rxAsdu.info.stream );(* Copy NVA value to local variable *)
				IF rxAsdu.ident.eType <> M_ME_ND_1 THEN
					F_iecMoveStreamToBuffer( ADR( stQds ), SIZEOF( stQds ), rxAsdu.info.stream );(* Copy QDS descriptor to local variable *)
					IF rxAsdu.ident.eType = M_ME_TA_1 THEN
						F_iecMoveStreamToBuffer( ADR( tT24 ), 3(* SIZEOF( tT24 ) - 1 *), rxAsdu.info.stream );(* Copy time tag to local variable *)
					ELSIF rxAsdu.ident.eType = M_ME_TD_1 THEN
						F_iecMoveStreamToBuffer( ADR( tT56 ), 7(* SIZEOF( tT56 ) - 1 *), rxAsdu.info.stream );(* Copy time tag to local variable *)
					END_IF
				END_IF
				IF rxAsdu.info.objAddr = 500 THEN
					stProcData.nNva500 := nNva;
					stProcData.stQds500 := stQds;
				END_IF
			(*-----------------------------------------------------------------------------------------*)
			M_ME_NB_1, M_ME_TB_1, M_ME_TE_1:(* Measured values, scaled values *)
				F_iecMoveStreamToBuffer( ADR( nSva ), SIZEOF( nSva ), rxAsdu.info.stream );(* Copy SVA value to local variable *)
				F_iecMoveStreamToBuffer( ADR( stQds ), SIZEOF( stQds ), rxAsdu.info.stream );(* Copy QDS descriptor to local variable *)
				IF rxAsdu.ident.eType = M_ME_TB_1 THEN
					F_iecMoveStreamToBuffer( ADR( tT24 ), 3(* SIZEOF( tT24 ) - 1 *), rxAsdu.info.stream );(* Copy time tag to local variable *)
				ELSIF rxAsdu.ident.eType = M_ME_TE_1 THEN
					F_iecMoveStreamToBuffer( ADR( tT56 ), 7(* SIZEOF( tT56 ) - 1 *), rxAsdu.info.stream );(* Copy time tag to local variable *)
				END_IF
				IF rxAsdu.info.objAddr = 600 THEN
					stProcData.nSva600 := nSva;
					stProcData.stQds600 := stQds;
				END_IF
			(*-----------------------------------------------------------------------------------------*)
			M_ME_NC_1, M_ME_TC_1, M_ME_TF_1:(* Measured values, short floating point value *)
				F_iecMoveStreamToBuffer( ADR( fR32 ), SIZEOF( fR32 ), rxAsdu.info.stream );(* Copy R32 value to local variable *)
				F_iecMoveStreamToBuffer( ADR( stQds ), SIZEOF( stQds ), rxAsdu.info.stream );(* Copy QDS descriptor to local variable *)
				IF rxAsdu.ident.eType = M_ME_TC_1 THEN
					F_iecMoveStreamToBuffer( ADR( tT24 ), 3(* SIZEOF( tT24 ) - 1 *), rxAsdu.info.stream );(* Copy time tag to local variable *)
				ELSIF rxAsdu.ident.eType = M_ME_TF_1 THEN
					F_iecMoveStreamToBuffer( ADR( tT56 ), 7(* SIZEOF( tT56 ) - 1 *), rxAsdu.info.stream );(* Copy time tag to local variable *)
				END_IF
				IF rxAsdu.info.objAddr = 700 THEN
					stProcData.fSingle700 := fR32;
					stProcData.stQds700 := stQds;
				END_IF
			(*-----------------------------------------------------------------------------------------*)
			M_IT_NA_1, M_IT_TA_1, M_IT_TB_1:(* Integrated totals *)
				F_iecMoveStreamToBuffer( ADR( nBcr ), SIZEOF( nBcr ), rxAsdu.info.stream );(* Copy BCR value to local variable *)
				F_iecMoveStreamToBuffer( ADR( stQcr ), SIZEOF( stQcr ), rxAsdu.info.stream );(* Copy QCR to local variable *)
				IF rxAsdu.ident.eType = M_IT_TA_1 THEN
					F_iecMoveStreamToBuffer( ADR( tT24 ), 3(* SIZEOF( tT24 ) - 1 *), rxAsdu.info.stream );(* Copy time tag to local variable *)
				ELSIF rxAsdu.ident.eType = M_IT_TB_1 THEN
					F_iecMoveStreamToBuffer( ADR( tT56 ), 7(* SIZEOF( tT56 ) - 1 *), rxAsdu.info.stream );(* Copy time tag to local variable *)
				END_IF 
				IF rxAsdu.info.objAddr = 800 THEN 
					stProcData.nBcr800	:= nBcr;
					stProcData.nQcr800 	:= stQcr;
				ELSIF rxAsdu.info.objAddr = 801 THEN 
					stProcData.nBcr801	:= nBcr;
					stProcData.nQcr801 	:= stQcr;
				ELSIF rxAsdu.info.objAddr = 802 THEN 
					stProcData.nBcr802	:= nBcr;
					stProcData.nQcr802 	:= stQcr;
				END_IF
			(*-----------------------------------------------------------------------------------------*)
			M_EP_TA_1, M_EP_TD_1:(* Events of protection equipment *)
				F_iecMoveStreamToBuffer( ADR( stSep ), SIZEOF( stSep ), rxAsdu.info.stream );(* Copy SEP value to local variable *)
				F_iecMoveStreamToBuffer( ADR( tT16 ), SIZEOF( tT16 ), rxAsdu.info.stream );(* Copy two octet time to local variable *)
				IF rxAsdu.ident.eType = M_EP_TA_1 THEN
					F_iecMoveStreamToBuffer( ADR( tT24 ), 3(* SIZEOF( tT24 ) - 1 *), rxAsdu.info.stream );(* Copy time tag to local variable *)
				ELSE
					F_iecMoveStreamToBuffer( ADR( tT56 ), 7(* SIZEOF( tT56 ) - 1 *), rxAsdu.info.stream );(* Copy time tag to local variable *)
				END_IF
			(*-----------------------------------------------------------------------------------------*)
			M_EP_TB_1, M_EP_TE_1:(* Packed start events of protection equipment *)
				F_iecMoveStreamToBuffer( ADR( stSpe ), SIZEOF( stSpe ), rxAsdu.info.stream );(* Copy SPE value to local variable *)
				F_iecMoveStreamToBuffer( ADR( stQdp ), SIZEOF( stQdp ), rxAsdu.info.stream );(* Copy QDP value to local variable *)
				F_iecMoveStreamToBuffer( ADR( tT16 ), SIZEOF( tT16 ), rxAsdu.info.stream );(* Copy two octet time to local variable *)
				IF rxAsdu.ident.eType = M_EP_TB_1 THEN
					F_iecMoveStreamToBuffer( ADR( tT24 ), 3(* SIZEOF( tT24 ) - 1 *), rxAsdu.info.stream );(* Copy time tag to local variable *)
				ELSE
					F_iecMoveStreamToBuffer( ADR( tT56 ), 7(* SIZEOF( tT56 ) - 1 *), rxAsdu.info.stream );(* Copy time tag to local variable *)
				END_IF
			(*-----------------------------------------------------------------------------------------*)
			M_EP_TC_1, M_EP_TF_1:(* Packed output circuit information of protection equipment *)
				F_iecMoveStreamToBuffer( ADR( stOci ), SIZEOF( stOci ), rxAsdu.info.stream );(* Copy OCI value to local variable *)
				F_iecMoveStreamToBuffer( ADR( stQdp ), SIZEOF( stQdp ), rxAsdu.info.stream );(* Copy QDP value to local variable *)
				F_iecMoveStreamToBuffer( ADR( tT16 ), SIZEOF( tT16 ), rxAsdu.info.stream );(* Copy two octet time to local variable *)
				IF rxAsdu.ident.eType = M_EP_TC_1 THEN
					F_iecMoveStreamToBuffer( ADR( tT24 ), 3(* SIZEOF( tT24 ) - 1 *), rxAsdu.info.stream );(* Copy time tag to local variable *)
				ELSE
					F_iecMoveStreamToBuffer( ADR( tT56 ), 7(* SIZEOF( tT56) - 1 *), rxAsdu.info.stream );(* Copy time tag to local variable *)
				END_IF
			(*-----------------------------------------------------------------------------------------*)
			M_PS_NA_1:(* Packed single point information with status change detection *)
				F_iecMoveStreamToBuffer( ADR( nScd ), SIZEOF( nScd ), rxAsdu.info.stream );(* Copy SCD value to local variable *)
				F_iecMoveStreamToBuffer( ADR( stQds ), SIZEOF( stQds ), rxAsdu.info.stream );(* Copy QDS value to local variable *)
			(*-----------------------------------------------------------------------------------------*)
			C_SC_NA_1, C_SC_TA_1:(* Single commands *)
				F_iecMoveStreamToBuffer( ADR( nSco ), SIZEOF( nSco ), rxAsdu.info.stream );(* Copy SCO value to local variable *)
				IF rxAsdu.ident.eType = C_SC_TA_1 THEN
					F_iecMoveStreamToBuffer( ADR( tT56 ), 7(* SIZEOF( tT56 ) - 1 *), rxAsdu.info.stream );(* Copy time tag to local variable *)
				END_IF
				IF rxAsdu.ident.eCOT = eIEC870_COT_ACT_CON THEN
					bCmdConWait := FALSE;(* Reset wait flag *)
				END_IF
				IF rxAsdu.ident.eCOT = eIEC870_COT_ACT_TERM THEN
					bCmdTermWait := FALSE;(* Reset wait flag *)
				END_IF
			(*-----------------------------------------------------------------------------------------*)
			C_DC_NA_1, C_DC_TA_1:(* Double commands *)
				F_iecMoveStreamToBuffer( ADR( nDco ), SIZEOF( nDco ), rxAsdu.info.stream );(* Copy DCO value to local variable *)
				IF rxAsdu.ident.eType = C_DC_TA_1 THEN
					F_iecMoveStreamToBuffer( ADR( tT56 ), 7(* SIZEOF( tT56 ) - 1*), rxAsdu.info.stream );(* Copy time tag to local variable *)
				END_IF
				IF rxAsdu.ident.eCOT = eIEC870_COT_ACT_CON THEN
					bCmdConWait := FALSE;(* Reset wait flag *)
				END_IF
				IF rxAsdu.ident.eCOT = eIEC870_COT_ACT_TERM THEN
					bCmdTermWait := FALSE;(* Reset wait flag *)
				END_IF
			(*-----------------------------------------------------------------------------------------*)
			C_RC_NA_1, C_RC_TA_1:(* Regulating step commands *)
				F_iecMoveStreamToBuffer( ADR( nRco ), SIZEOF( nRco ), rxAsdu.info.stream );(* Copy RCO value to local variable *)
				IF rxAsdu.ident.eType = C_RC_TA_1 THEN
					F_iecMoveStreamToBuffer( ADR( tT56 ), 7(* SIZEOF( tT56 ) - 1 *), rxAsdu.info.stream );(* Copy time tag to local variable *)
				END_IF
				IF rxAsdu.ident.eCOT = eIEC870_COT_ACT_CON THEN
					bCmdConWait := FALSE;(* Reset wait flag *)
				END_IF
				IF rxAsdu.ident.eCOT = eIEC870_COT_ACT_TERM THEN
					bCmdTermWait := FALSE;(* Reset wait flag *)
				END_IF
			(*-----------------------------------------------------------------------------------------*)
			C_SE_NA_1,C_SE_TA_1:(* Setpoint commands, normalized values *)
				F_iecMoveStreamToBuffer( ADR( nNva ), SIZEOF( nNva ), rxAsdu.info.stream );(* Copy NVA value to local variable *)
				F_iecMoveStreamToBuffer( ADR( nQos ), SIZEOF( nQos ), rxAsdu.info.stream );(* Copy QOS value to local variable *)
				IF rxAsdu.ident.eType = C_SE_TA_1 THEN
					F_iecMoveStreamToBuffer( ADR( tT56 ), 7(* SIZEOF( tT56 ) - 1 *), rxAsdu.info.stream );(* Copy time tag to local variable *)
				END_IF
				IF rxAsdu.ident.eCOT = eIEC870_COT_ACT_CON THEN
					bCmdConWait := FALSE;(* Reset wait flag *)
				END_IF
				IF rxAsdu.ident.eCOT = eIEC870_COT_ACT_TERM THEN
					bCmdTermWait := FALSE;(* Reset wait flag *)
				END_IF
			(*-----------------------------------------------------------------------------------------*)
			C_SE_NB_1, C_SE_TB_1:(* Setpoint commands, scaled values *)
				F_iecMoveStreamToBuffer( ADR( nSva ), SIZEOF( nSva ), rxAsdu.info.stream );(* Copy SVA value to local variable *)
				F_iecMoveStreamToBuffer( ADR( nQos ), SIZEOF( nQos ), rxAsdu.info.stream );(* Copy QOS value to local variable *)
				IF rxAsdu.ident.eType = C_SE_TB_1 THEN
					F_iecMoveStreamToBuffer( ADR( tT56 ), 7(* SIZEOF( tT56 ) - 1 *), rxAsdu.info.stream );(* Copy time tag to local variable *)
				END_IF
				IF rxAsdu.ident.eCOT = eIEC870_COT_ACT_CON THEN
					bCmdConWait := FALSE;(* Reset wait flag *)
				END_IF
				IF rxAsdu.ident.eCOT = eIEC870_COT_ACT_TERM THEN
					bCmdTermWait := FALSE;(* Reset wait flag *)
				END_IF
			(*-----------------------------------------------------------------------------------------*)
			C_SE_NC_1, C_SE_TC_1:(* Setpoint commands, short floating point values *)
				F_iecMoveStreamToBuffer( ADR( fR32 ), SIZEOF( fR32 ), rxAsdu.info.stream );(* Copy R32 value to local variable *)
				F_iecMoveStreamToBuffer( ADR( nQos ), SIZEOF( nQos ), rxAsdu.info.stream );(* Copy QOS value to local variable *)
				IF rxAsdu.ident.eType = C_SE_TC_1 THEN
					F_iecMoveStreamToBuffer( ADR( tT56 ), 7(* SIZEOF( tT56 ) - 1 *), rxAsdu.info.stream );(* Copy time tag to local variable *)
				END_IF
				IF rxAsdu.ident.eCOT = eIEC870_COT_ACT_CON THEN
					bCmdConWait := FALSE;(* Reset wait flag *)
				END_IF
				IF rxAsdu.ident.eCOT = eIEC870_COT_ACT_TERM THEN
					bCmdTermWait := FALSE;(* Reset wait flag *)
				END_IF
			(*-----------------------------------------------------------------------------------------*)
			C_BO_NA_1, C_BO_TA_1:(* Bistring commands *)
				F_iecMoveStreamToBuffer( ADR( nBsi ), SIZEOF( nBsi ), rxAsdu.info.stream );(* Copy BSI value to local variable *)
				IF rxAsdu.ident.eType = C_BO_TA_1 THEN
					F_iecMoveStreamToBuffer( ADR( tT56 ), 7(* SIZEOF( tT56 ) - 1 *), rxAsdu.info.stream );(* Copy time tag to local variable *)
				END_IF
				IF rxAsdu.ident.eCOT = eIEC870_COT_ACT_CON THEN
					bCmdConWait := FALSE;(* Reset wait flag *)
				END_IF
				IF rxAsdu.ident.eCOT = eIEC870_COT_ACT_TERM THEN(* Optional *)
					bCmdTermWait := FALSE;(* Reset wait flag *)
				END_IF
			(*-----------------------------------------------------------------------------------------*)
			M_EI_NA_1:(* End of initialization *)
				F_iecMoveStreamToBuffer( ADR( nCoi ), SIZEOF( nCoi ), rxAsdu.info.stream );(* Copy COI to local variable *)
				eCoi := nCoi AND 2#1111111;
				bLpc := nCoi.7;
			(*-----------------------------------------------------------------------------------------*)
			C_RD_NA_1:(* Read data command *)
				(* TODO... *);
			(*-----------------------------------------------------------------------------------------*)
			C_RP_NA_1:(* Reset process command *)
				IF rxAsdu.ident.eCOT = eIEC870_COT_ACT_CON THEN
					bCmdConWait := FALSE;(* Reset wait flag *)
				END_IF
			(*-----------------------------------------------------------------------------------------*)
			P_ME_NA_1:(* Parameter of measured value, normalized value *)
				F_iecMoveStreamToBuffer( ADR( nNva ), SIZEOF( nNva ), rxAsdu.info.stream );(* Copy NVA value to local variable *)
				F_iecMoveStreamToBuffer( ADR( nQpm ), SIZEOF( nQpm ), rxAsdu.info.stream );(* Copy QPM to local variable *)
			(*-----------------------------------------------------------------------------------------*)
			P_ME_NB_1:(* Parameter of measured value, scaled value *)
				F_iecMoveStreamToBuffer( ADR( nSva ), SIZEOF( nSva ), rxAsdu.info.stream );(* Copy SVA value to local variable *)
				F_iecMoveStreamToBuffer( ADR( nQpm ), SIZEOF( nQpm ), rxAsdu.info.stream );(* Copy QPM to local variable *)
			(*-----------------------------------------------------------------------------------------*)
			P_ME_NC_1:(* Parameter of measured value, short floating point value *)
				F_iecMoveStreamToBuffer( ADR( fR32 ), SIZEOF( fR32 ), rxAsdu.info.stream );(* Copy R32 value to local variable *)
				F_iecMoveStreamToBuffer( ADR( nQpm ), SIZEOF( nQpm ), rxAsdu.info.stream );(* Copy QPM to local variable *)
			(*-----------------------------------------------------------------------------------------*)
			P_AC_NA_1:(* Parameter activation *)
				F_iecMoveStreamToBuffer( ADR( nQpa ), SIZEOF( nQpa ), rxAsdu.info.stream );(* Copy QPA to local variable *)

		ELSE(* Report invalid asdu type...*)
			fbLog.A_LogError( sPut := '::Unsupported asdu type!' );
			EXIT;
		END_CASE

	END_IF
UNTIL NOT fbBuffer.bOk (* RX fifo is empty *)
END_REPEAT

END_FUNCTION_BLOCK
